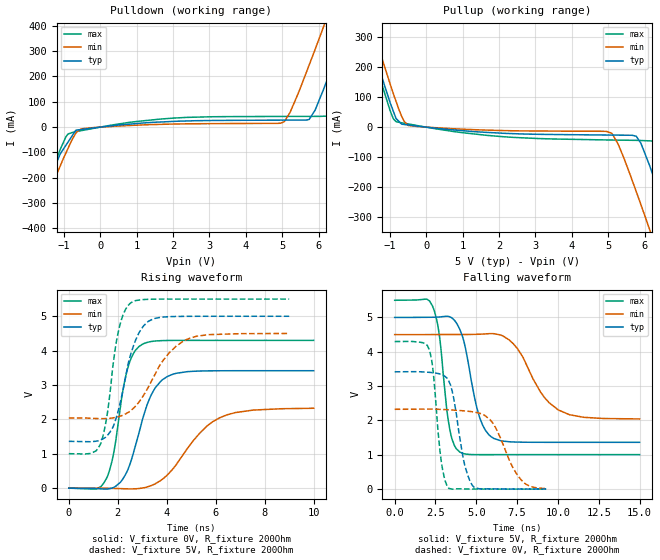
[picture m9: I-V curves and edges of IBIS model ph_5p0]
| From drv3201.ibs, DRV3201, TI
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|   ph_5p0 Model
[Model]   ph_5p0
Model_type   Output
Polarity   Non-Inverting
Vmeas = 2.5
Vref = 0
Cref = 2pF
Rref = 300
|   typ   min   max
|   (nom PVT)   (fast PVT)   (slow PVT)
C_comp   1.397e-12   1.378e-12   1.437e-12
| Where nom  PVT is Nominal Process, 5V, 27C
|   Fast PVT is Strong Process,  5.5V, -40C
|   Slow PVT is Weak Process,   4.5V, 150C
[Voltage Range]   5   4.5   5.5
|Junction Temperature
[Temperature Range]   27   150   -40
[Pullup Reference]   5   4.5   5.5
[Pulldown Reference]   0   0   0
[Power Clamp Reference]   5   4.5   5.5
[GND Clamp Reference]   0   0   0
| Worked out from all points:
|   slope of the pulldown table from 0 to 0.75 V, typ, clamps not added: 66.9 ohm
|   slope of the pullup table from 0 to 0.75 V, typ, clamps not added: 81.7 ohm
|   falling waveform, V_fixture 5V, R_fixture 200Ohm: 20-80 % time 947ps typ, 1.79ns min, 619ps max; typ from 5 V to 1.36 V
|   rising waveform, V_fixture 0V, R_fixture 200Ohm: 20-80 % time 891ps typ, 1.6ns min, 601ps max; typ from 0 V to 3.42 V
|   rising waveform, V_fixture 5V, R_fixture 200Ohm: 20-80 % time 754ps typ, 1.31ns min, 529ps max; typ from 1.36 V to 5 V
|   falling waveform, V_fixture 0V, R_fixture 200Ohm: 20-80 % time 721ps typ, 1.34ns min, 486ps max; typ from 3.42 V to 0 V
[Pulldown]
|   Voltage   I(typ)   I(min)   I(max)
-5V       -1.602A    -1.591A    -1.636A
-1.985V   -429.3mA   -467.8mA   -427.2mA
-951.5mV  -73.59mA   -104.9mA   -40.93mA
-526.5mV  -9.525mA   -6.961mA   -13.93mA
2.041V    22.84mA    12.23mA    35.89mA
5.049V    27.67mA    20.74mA    42.31mA
5.74V     30.36mA    245.2mA    42.48mA
6.13V     146.9mA    394.1mA    42.98mA
6.407V    252.2mA    502.3mA    53.84mA
6.835V    419.3mA    670.4mA    205.3mA
8.14V     940.3mA    1.191A     724.9mA
10V       1.695A     1.934A     1.485A
[Pullup]
|   Voltage   I(typ)   I(min)   I(max)
-5V       1.71A      1.748A     1.703A
-2.535V   698.9mA    752mA      680.4mA
-1.375V   230mA      291.3mA    204.3mA
-891mV    50mA       108.3mA    26.5mA
-486mV    7.103mA    5.491mA    10.56mA
5.098V    -26.46mA   -20.2mA    -43.03mA
5.775V    -30.49mA   -215.8mA   -44.05mA
6.129V    -124.5mA   -337.3mA   -45.71mA
6.407V    -220.4mA   -435.7mA   -52.97mA
6.835V    -374.1mA   -588.7mA   -189.5mA
7.843V    -752.2mA   -957.3mA   -570mA
10V       -1.587A    -1.765A    -1.423A
[Ramp]
R_load = 200
|   typ   min   max
dV/dt_r   2.04946/8.89608e-10   1.39444/1.59904e-09   2.57904/5.97685e-10
dV/dt_f   2.1827/9.46291e-10   1.47426/1.77761e-09   2.69829/6.13721e-10
[Falling Waveform]
V_fixture = 5V
V_fixture_min = 4.5V
V_fixture_max = 5.5V
R_fixture = 200Ohm
|   Time   V(typ)   V(min)   V(max)
0s        5V         4.5V       5.5V
2.318ns   5.006V     4.501V     5.332V
2.742ns   5.014V     4.502V     4.461V
3.368ns   5.02V      4.502V     1.756V
3.996ns   4.645V     4.503V     1.077V
5.198ns   2.095V     4.511V     1.003V
6.074ns   1.474V     4.527V     1.003V
7.51ns    1.368V     4.098V     1.003V
10.03ns   1.362V     2.304V     1.003V
15ns      1.362V     2.043V     1.003V
[Rising Waveform]
V_fixture = 0V
V_fixture_min = 0V
V_fixture_max = 0V
R_fixture = 200Ohm
|   Time   V(typ)   V(min)   V(max)
0s        1.081nV    205.8nV    828.7pV
1.106ns   -11.69mV   1.278mV    -26.99mV
1.532ns   -29.01mV   -2.975mV   274.1mV
1.822ns   17.29mV    -7.79mV    976.6mV
2.402ns   517.3mV    -20.84mV   3.478V
3.004ns   1.985V     3.265mV    4.184V
3.55ns    2.937V     134.2mV    4.281V
4.272ns   3.319V     577.8mV    4.298V
6.158ns   3.414V     2.046V     4.298V
9.998ns   3.416V     2.324V     4.298V
[Rising Waveform]
V_fixture = 5V
V_fixture_min = 4.5V
V_fixture_max = 5.5V
R_fixture = 200Ohm
|   Time   V(typ)   V(min)   V(max)
0s        1.362V     2.041V     1.003V
1.31ns    1.406V     2.022V     1.301V
1.582ns   1.538V     2.027V     2.206V
1.994ns   2.184V     2.071V     4.451V
2.206ns   2.823V     2.121V     5.021V
2.544ns   3.93V      2.264V     5.396V
3.258ns   4.857V     2.951V     5.493V
3.874ns   4.978V     3.738V     5.499V
4.804ns   4.998V     4.32V      5.5V
8.998ns   5V         4.5V       5.5V
[Falling Waveform]
V_fixture = 0V
V_fixture_min = 0V
V_fixture_max = 0V
R_fixture = 200Ohm
|   Time   V(typ)   V(min)   V(max)
0s        3.416V     2.324V     4.298V
2.098ns   3.401V     2.33V      4.082V
2.368ns   3.388V     2.328V     3.375V
2.854ns   3.34V      2.32V      802.5mV
3.324ns   3.138V     2.309V     18.16mV
4.198ns   894.3mV    2.28V      3.89mV
4.758ns   105.5mV    2.252V     288.4uV
6.028ns   4.949mV    1.909V     -37.38uV
7.888ns   81.72uV    196.3mV    69.66nV
9.278ns   7.471uV    13.24mV    -115.6nV
